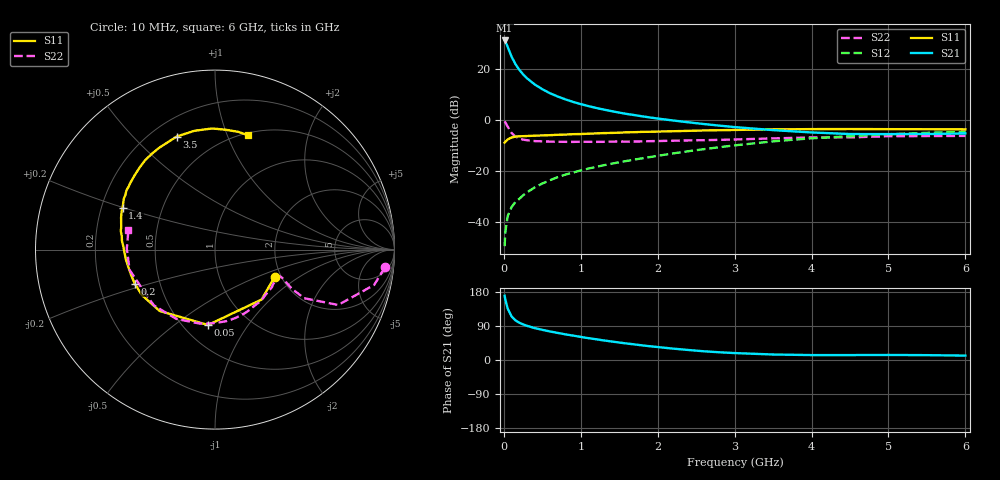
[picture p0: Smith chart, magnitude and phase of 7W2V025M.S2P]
! Infineon Technologies  Discrete & RF Semiconductors
! BFS17W
! Si NPN RF Bipolar Junction Transistor in SOT323
! VCE = 2 V  IC = 25 mA
! Common Emitter S-Parameters:  August  1999
# GHz  S  MA  R  50
!  f  S11  S21  S12  S22
! GHz  MAG  ANG  MAG  ANG  MAG  ANG  MAG  ANG
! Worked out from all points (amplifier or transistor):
!   36 points, 10 MHz to 6 GHz, reference 50 ohm
!   highest |S21| = 31.3 dB at 10 MHz (marker M1)
!   |S21| within 3 dB of that: start of sweep to 56.25 MHz
!   unconditionally stable (mu >= 1): 192.3 MHz to 3.107 GHz; 3.654 GHz to end of sweep
!   at 250 MHz: K = 1.11, MAG = 21.7 dB, |S12| = -29.4 dB
!   at 1.4 GHz: K = 1.26, MAG = 7.2 dB, |S12| = -17.0 dB
!   at 6 GHz: K = 1.10, MAG = -2.3 dB, |S12| = -4.4 dB
!   S11 on the Smith chart (normalised r, x): 10 MHz: 1.84, -0.65; 50 MHz: 0.65, -0.67; 200 MHz: 0.36, -0.18; 1.4 GHz: 0.29, +0.20; 3.5 GHz: 0.30, +0.67; 6 GHz: 0.52, +1.19
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0.01  0.3655 -24.8  36.83 169.6  0.0034 81.1  0.9516 -6.0
0.02  0.3804 -47.1  35.18 159.1  0.0065 79.6  0.9085 -12.5
0.05  0.4218 -95.3  27.53 135.5  0.0133 64.7  0.7524 -24.2
0.1  0.4603 -132.0  17.81 115.2  0.0198 58.9  0.5657 -28.6
0.15  0.4798 -148.1  12.74 104.8  0.0249 58.4  0.4808 -27.0
0.2  0.4857 -157.0  9.838 98.5  0.0288 61.9  0.4418 -25.0
0.25  0.4884 -163.3  7.973 93.9  0.0337 62.7  0.4184 -23.5
0.3  0.4913 -167.4  6.69 90.2  0.0385 65.4  0.4068 -22.8
0.4  0.5 -173.9  5.071 84.3  0.0482 66.8  0.3915 -22.4
0.5  0.5052 -178.5  4.074 79.6  0.0576 68.9  0.3864 -23.0
0.6  0.5111 178.0  3.397 75.3  0.0669 69.3  0.3824 -24.4
0.7  0.5203 174.9  2.931 71.5  0.0766 70.1  0.3798 -26.4
0.9  0.5347 169.0  2.297 64.4  0.0944 70.5  0.377 -31.1
1.1  0.5464 163.2  1.898 57.6  0.113 70.5  0.3786 -36.8
1.4  0.5654 155.6  1.512 48.9  0.1406 70.5  0.3821 -46.3
1.8  0.5935 146.2  1.196 38.5  0.1799 70.1  0.3865 -59.9
2.2  0.6105 136.9  0.992 30.0  0.2242 68.7  0.3979 -73.7
2.8  0.6392 123.4  0.787 20.4  0.2966 64.3  0.4136 -95.0
3.5  0.6649 108.8  0.642 14.5  0.3865 56.7  0.4421 -119.2
4.5  0.6749 91.3  0.538 13.0  0.4873 43.2  0.4619 -153.3
5.5  0.6688 78.9  0.538 12.8  0.568 30.9  0.4914 179.4
6  0.6636 74.1  0.553 11.6  0.5999 25.2  0.4944 167.4
